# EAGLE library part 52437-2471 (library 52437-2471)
FFC & FPC Connectors RA SMT ZIF BTTM 24P GOLD Source: Datasheet
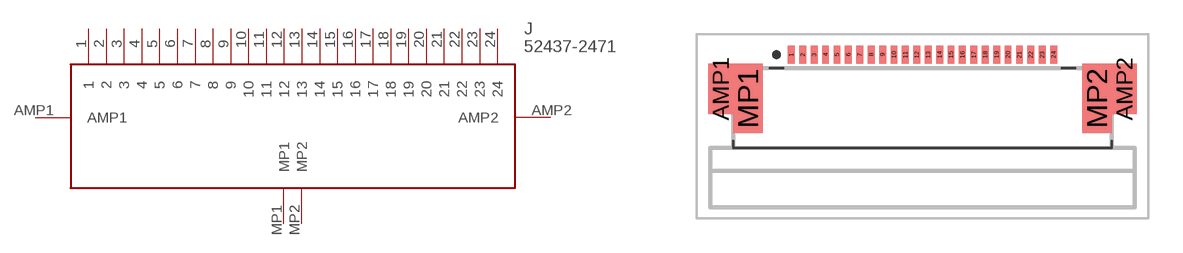
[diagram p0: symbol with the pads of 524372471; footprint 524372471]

Designator prefix J

## 52437-2471 (Description: FFC & FPC Connectors RA SMT ZIF BTTM 24P GOLD; Height: 2mm; Manufacturer_Name: Molex; Manufacturer_Part_Number: 52437-2471; Mouser_Part_Number: 538-52437-2471; Mouser_Price-Stock: https://www.mouser.co.uk/ProductDetail/Molex/52437-2471?qs=nDwhpid8gJZdpyQIeZfjsA%3D%3D)  [524372471]
1  1
2  2
3  3
4  4
5  5
6  6
7  7
8  8
9  9
10  10
11  11
12  12
13  13
14  14
15  15
16  16
17  17
18  18
19  19
20  20
21  21
22  22
23  23
24  24
AMP1  AMP1
AMP2  AMP2
MP1  MP1
MP2  MP2

## Footprint 524372471 (pad centres in mm)
52437-2471-1
smd 0.3 x 0.8: 1 -5.75,3.15; 2 -5.25,3.15; 3 -4.75,3.15; 4 -4.25,3.15; 5 -3.75,3.15; 6 -3.25,3.15; 7 -2.75,3.15; 8 -2.25,3.15; 9 -1.75,3.15; 10 -1.25,3.15; 11 -0.75,3.15; 12 -0.25,3.15; 13 0.25,3.15; 14 0.75,3.15; 15 1.25,3.15; 16 1.75,3.15; 17 2.25,3.15; 18 2.75,3.15; 19 3.25,3.15; 20 3.75,3.15; 21 4.25,3.15; 22 4.75,3.15; 23 5.25,3.15; 24 5.75,3.15
smd 1.1 x 2.2: AMP1 -8.85,1.65; AMP2 8.85,1.65
smd 1.3 x 3.05: MP1 -7.65,1.225; MP2 7.65,1.225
